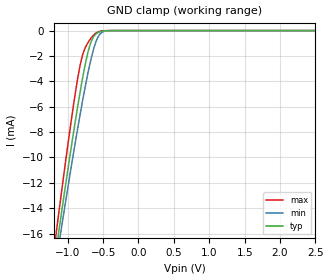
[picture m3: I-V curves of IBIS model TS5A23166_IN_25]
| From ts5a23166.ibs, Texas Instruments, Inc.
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[Model]   TS5A23166_IN_25
Model_type  Input
Vinl=0.6
Vinh=1.8
| variable   typ   min   max
C_comp   1.64pF   1.35pF   1.98pF
[Temperature Range]   40   100   -40
| Ambient temperature   25   85   -40
[Voltage range]   2.5   2.3   2.7
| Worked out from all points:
|   GND clamp passes 1 mA (typ) near -0.68 V on its own axis
[GND Clamp]
| TS5A23166_IN_25
|   Voltage   I(typ)   I(min)   I(max)
-2.5V     -73.44mA   -69.94mA   -77.66mA
-1.175V   -17.77mA   -18.67mA   -16.5mA
-1.15V    -16.79mA   -17.77mA   -15.42mA
-1.125V   -15.81mA   -16.87mA   -14.34mA
-1.085V   -14.27mA   -15.45mA   -12.64mA
-925mV    -8.305mA   -9.904mA   -6.147mA
-820mV    -4.705mA   -6.482mA   -2.626mA
-770mV    -3.17mA    -4.953mA   -1.604mA
-695mV    -1.321mA   -2.864mA   -792.2uA
-590mV    -223.9uA   -735.2uA   -163.6uA
-425mV    -5.378uA   -12.34uA   -1.336uA
2.5V      44.8pA     113.3pA    30.06pA
